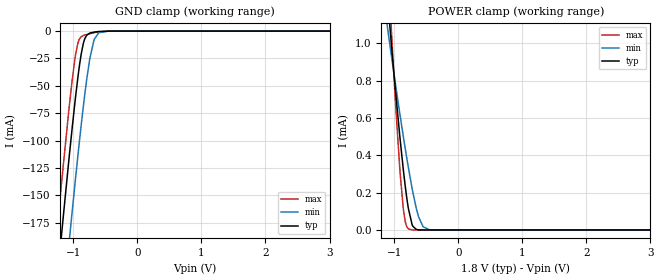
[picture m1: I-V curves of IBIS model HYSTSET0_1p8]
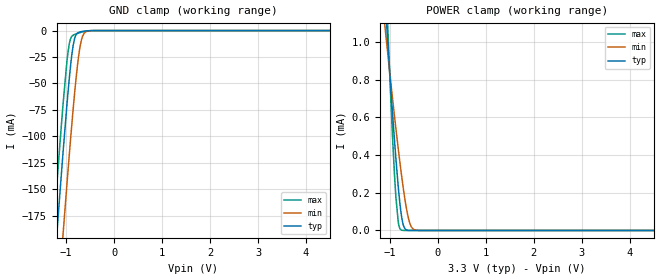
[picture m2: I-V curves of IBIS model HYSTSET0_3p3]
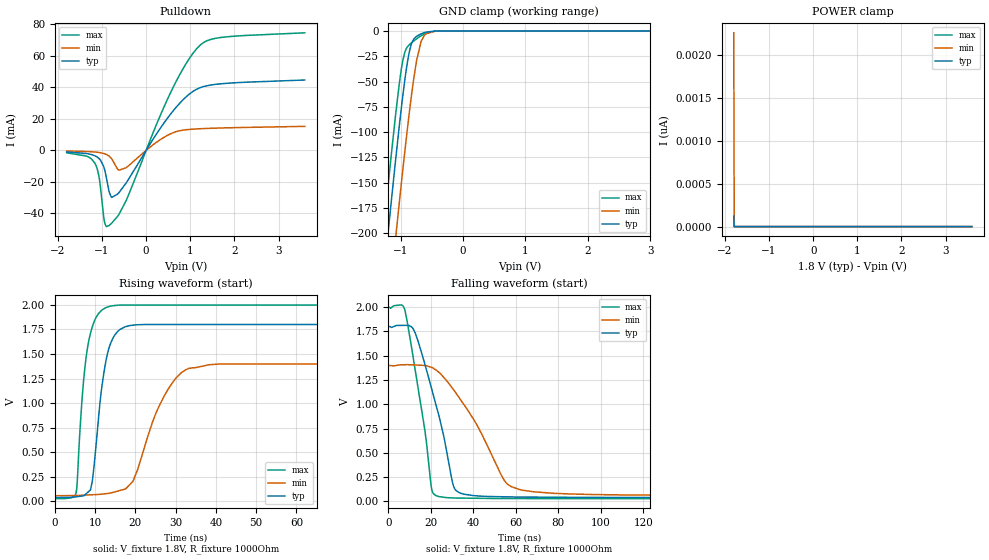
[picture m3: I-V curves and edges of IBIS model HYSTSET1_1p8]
|Texas Instruments Incorporated
| Marketing part#   Digital Voltage Range   Package-type   #pins
|  TMP303A/B/C   1.4V - 3.6V   SOT   6
[IBIS Ver]   4.1
[File name]   tmp303.ibs
[File Rev]   1.0
[Date]   11/03/2015
[Source]
| Texas Instruments Incorporated.
| 12500 TI Blvd
| Dallas, TX -75243
[Notes]   Revision History:
| Rev 1.0: 11/03/2015
| - Initial version of the model
| - Model generated from simulations in TISPICE
| - C_comp although listed in numerical order of value are
|   obtained from varying PVT conditions. For PVT conditions for
|   each specific value refer the buffer description under
|   respective [Model]. IBIS model user is responsible for using
|   appropriate C_comp to simulate for Signal Integrity.
| - Warnings regarding combined Non-monotonicity of various models have been
|   reviewd and considered minor and can be ignored.
| - Model names with a trailing _1p8 contain the model for
|   1.8V operation. Model names with a trailing _3p3 contain the model
|   for 3.3V operation.
[Disclaimer]
| This model is designed as an aid for customers of Texas Instruments.
| TI and its licensors and suppliers make no warranties, either expressed
| or implied, with respect to this  model, including the warranties of
| merchantability or fitness for a particular purpose. The model is
| provided solely on an "as is" basis. The entire risk as to its quality
| and performance is with the customer.
[Copyright]
 (C) Copyright 2015 Texas Instruments Incorporated.All rights reserved.
|   Device
[Component]  TMP303
[Manufacturer]   TI
[Package]
| variable   typ   min   max
R_pkg   0.2   0.16   0.24
L_pkg   1.5nH   1.2nH   1.8nH
C_pkg   0.4pF   0.32pF   0.48pF
[Pin]  signal_name   model_name   R_pin   L_pin   C_pin
1   HYST_SET0   HYSTSET0   NA   NA   NA
2   GND   GND   NA   NA   NA
3   OUT   OUT   NA   NA   NA
4   SOH   SOH   NA   NA   NA
5   VS   POWER   NA   NA   NA
6   HYST_SET1   HYSTSET1   NA   NA   NA
|   Model Selectors
[Model Selector]  HYSTSET0
HYSTSET0_3p3  HYSTSET0 buffer at 3.3V operation.
HYSTSET0_1p8  HYSTSET0 buffer at 1.8V operation.
[Model Selector]  HYSTSET1
HYSTSET1_3p3  HYSTSET1 buffer at 3.3V operation.
HYSTSET1_1p8  HYSTSET1 buffer at 1.8V operation.
[Model Selector]  OUT
OUT_3p3  OUT buffer at 3.3V operation.
OUT_1p8  OUT buffer at 1.8V operation.
[Model Selector]  SOH
SOH_3p3  SOH buffer at 3.3V operation.
SOH_1p8  SOH buffer at 1.8V operation.
| Models and submodels in the file (8): HYSTSET0_1p8 (Input), HYSTSET0_3p3 (Input), HYSTSET1_1p8 (I/O_open_drain), HYSTSET1_3p3 (I/O_open_drain), OUT_1p8 (Output), OUT_3p3 (Output), SOH_1p8 (Input), SOH_3p3 (Input)
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|   Model
[Model]   HYSTSET0_1p8
Model_type   Input
Vinl = 0.54
Vinh = 1.26
|   typ   min   max
C_comp   1pF   1pF   1pF
[Voltage Range]   1.8   1.4   2
[Temperature Range]   25   125   -40
[Power Clamp Reference]   1.8   1.4   2
[GND Clamp Reference]   -0   -0   -0
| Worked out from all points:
|   GND clamp passes 1 mA (typ) near -0.68 V on its own axis
|   POWER clamp passes 1 mA (typ) near -1.04 V on its own axis
[GND Clamp]
|   Voltage   I(typ)   I(min)   I(max)
-1.8V     -577.8mA   -655.1mA   -532mA
-1.433V   -342mA     -420.5mA   -295.2mA
-1.217V   -206.8mA   -285.4mA   -159.7mA
-1.184V   -186.9mA   -265.4mA   -139.9mA
-1.066V   -116.1mA   -193.5mA   -70.51mA
-963mV    -59.55mA   -133.7mA   -21.17mA
-876.6mV  -21.18mA   -86.19mA   -5.211mA
-817.2mV  -6.6mA     -56.42mA   -3.572mA
-741.6mV  -1.819mA   -25.03mA   -2.385mA
-676.8mV  -927.9uA   -8.277mA   -1.52mA
-601.2mV  -384uA     -1.493mA   -702.1uA
3.595V    0A         0A         0A
[POWER Clamp]
|   Voltage   I(typ)   I(min)   I(max)
-1.8V     4.221mA    2.885mA    6.358mA
-1.179V   1.54mA     1.269mA    1.957mA
-1.028V   932.4uA    896.8uA    972.7uA
-968.4mV  707uA      755.2uA    623.2uA
-903.6mV  475.8uA    605.2uA    292.8uA
-849.6mV  301.2uA    484.8uA    95.08uA
-779.4mV  117.4uA    336.9uA    6.112uA
-714.6mV  24.29uA    213.3uA    255.9nA
-617.4mV  717.1nA    69.43uA    0A
-547.2mV  44nA       17.1uA     0A
-450mV    0A         1.247uA    0A
3.595V    0A         0A         0A
|   Model
[Model]   HYSTSET0_3p3
Model_type   Input
Vinl = 0.99
Vinh = 2.31
|   typ   min   max
C_comp   1pF   1pF   1pF
[Voltage Range]   3.3   2.7   3.6
[Temperature Range]   25   125   -40
[Power Clamp Reference]   3.3   2.7   3.6
[GND Clamp Reference]   -0   -0   -0
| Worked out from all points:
|   GND clamp passes 1 mA (typ) near -0.68 V on its own axis
|   POWER clamp passes 1 mA (typ) near -1.04 V on its own axis
[GND Clamp]
|   Voltage   I(typ)   I(min)   I(max)
-3.3V     -1.561A    -1.634A    -1.518A
-1.31V    -264.7mA   -343.3mA   -217.6mA
-1.261V   -233.8mA   -312.5mA   -186.7mA
-1.191V   -191.2mA   -269.7mA   -144.1mA
-1.063V   -114.4mA   -191.7mA   -68.86mA
-963.6mV  -59.86mA   -134mA     -21.39mA
-914.1mV  -36.09mA   -106.3mA   -8.588mA
-854.7mV  -14.34mA   -74.86mA   -4.398mA
-735.9mV  -1.702mA   -23.11mA   -2.304mA
-656.7mV  -752.6uA   -5.393mA   -1.279mA
-508.2mV  -78.78uA   -190.4uA   -136.9uA
6.59V     0A         0A         0A
[POWER Clamp]
|   Voltage   I(typ)   I(min)   I(max)
-3.3V     10.72mA    6.889mA    16.57mA
-1.092V   1.189mA    1.055mA    1.385mA
-1.023V   915.7uA    886uA      947.1uA
-943.8mV  618.8uA    698.4uA    492.7uA
-874.5mV  380.5uA    540.4uA    175.8uA
-825mV    230.9uA    432.3uA    43.68uA
-755.7mV  73.48uA    290.5uA    1.989uA
-706.2mV  18.77uA    199uA      167.9nA
-617.1mV  713.3nA    69.34uA    0A
-547.8mV  42.8nA     17.42uA    0A
-468.6mV  0A         2.121uA    0A
6.59V     0A         0A         0A
|   Model
[Model]   HYSTSET1_1p8
Model_type   I/O_open_drain
Polarity   Non-Inverting
Enable   Active-Low
Vinl = 0.54
Vinh = 1.26
Vmeas = 0.9
Vref = 1.8
Cref = 1pF
Rref = 1000
|   typ   min   max
C_comp   1pF   1pF   1pF
[Voltage Range]   1.8   1.4   2
[Temperature Range]   25   125   -40
[Pullup Reference]   1.8   1.4   2
[Pulldown Reference]   -0   -0   -0
[Power Clamp Reference]   1.8   1.4   2
[GND Clamp Reference]   -0   -0   -0
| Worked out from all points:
|   slope of the pulldown table from 0 to 0.27 V, typ, clamps not added: 22.7 ohm
|   GND clamp passes 1 mA (typ) near -0.58 V on its own axis
|   falling waveform, V_fixture 1.8V, R_fixture 1000Ohm: 20-80 % time 11.7ns typ, 20.6ns min, 8.07ns max; typ from 1.8 V to 0.038 V
|   rising waveform, V_fixture 1.8V, R_fixture 1000Ohm: 20-80 % time 2.96ns typ, 7.41ns min, 2.45ns max; typ from 0.038 V to 1.8 V
[Pulldown]
|   Voltage   I(typ)   I(min)   I(max)
-1.8V     -961.5uA   -381.3uA   -1.508mA
-1.157V   -3.463mA   -1.04mA    -8.218mA
-1.066V   -5.182mA   -1.34mA    -16.96mA
-930.6mV  -13.28mA   -2.209mA   -46.8mA
-838.8mV  -26.33mA   -3.588mA   -47.64mA
-774mV    -29.75mA   -5.568mA   -45.92mA
-617.4mV  -26.86mA   -12.57mA   -40.69mA
532.8mV   22.25mA    10.23mA    35.39mA
900mV     33.8mA     13.08mA    54.79mA
1.213V    39.66mA    13.73mA    66.45mA
1.71V     42.28mA    14.23mA    71.67mA
3.595V    44.65mA    15.25mA    74.57mA
[GND Clamp]
|   Voltage   I(typ)   I(min)   I(max)
-1.8V     -578.2mA   -655.5mA   -532.5mA
-1.233V   -217.6mA   -296mA     -171mA
-1.19V    -191.2mA   -269.5mA   -144.7mA
-1.082V   -126.8mA   -204mA     -82.07mA
-990mV    -75.61mA   -150.2mA   -37.17mA
-936mV    -48.67mA   -119.7mA   -21.09mA
-849.6mV  -17.04mA   -73.9mA    -12.76mA
-747mV    -5.205mA   -29.33mA   -7.75mA
-676.8mV  -2.855mA   -10.87mA   -4.788mA
-628.2mV  -1.718mA   -4.785mA   -3.02mA
-450mV    -55.33uA   -146.7uA   -73.73uA
3.595V    0A         0A         0A
[POWER Clamp]
|   Voltage   I(typ)   I(min)   I(max)
-1.8V     122.9pA    2.258nA    85.96pA
-1.789V   0A         0A         0A
-1.784V   0A         0A         0A
3.595V    0A         0A         0A
[Ramp]
R_load = 1000
|   typ   min   max
dV/dt_r   1.05701/2.95661e-09   0.805467/7.41211e-09   1.18366/2.44691e-09
dV/dt_f   1.05701/1.17501e-08   0.805467/2.06146e-08   1.18366/8.07842e-09
[Falling Waveform]
V_fixture = 1.8V
V_fixture_min = 1.4V
V_fixture_max = 2V
R_fixture = 1000Ohm
C_fixture = 0F
|   Time   V(typ)   V(min)   V(max)
0s        1.8V       1.4V       2V
7.679ns   1.812V     1.407V     1.978V
12.45ns   1.744V     1.404V     1.381V
20.48ns   1.152V     1.379V     118.6mV
26.95ns   575.4mV    1.255V     39.51mV
30.68ns   158.3mV    1.15V      34.98mV
33.28ns   90.92mV    1.069V     33.81mV
55.79ns   46.32mV    183.9mV    29.04mV
77.75ns   42.39mV    82.81mV    28.18mV
1us       38.31mV    57.55mV    27.23mV
[Rising Waveform]
V_fixture = 1.8V
V_fixture_min = 1.4V
V_fixture_max = 2V
R_fixture = 1000Ohm
C_fixture = 0F
|   Time   V(typ)   V(min)   V(max)
0s        38.31mV    57.55mV    27.23mV
5.318ns   46.62mV    59.33mV    91.19mV
7.08ns    56.67mV    62.92mV    1.194V
8.883ns   117.9mV    66.59mV    1.714V
12.64ns   1.417V     78.3mV     1.972V
16.15ns   1.749V     110.5mV    1.999V
19.42ns   1.794V     204.4mV    1.999V
29.64ns   1.801V     1.232V     1.999V
40.92ns   1.801V     1.399V     1.999V
1us       1.8V       1.4V       2V
